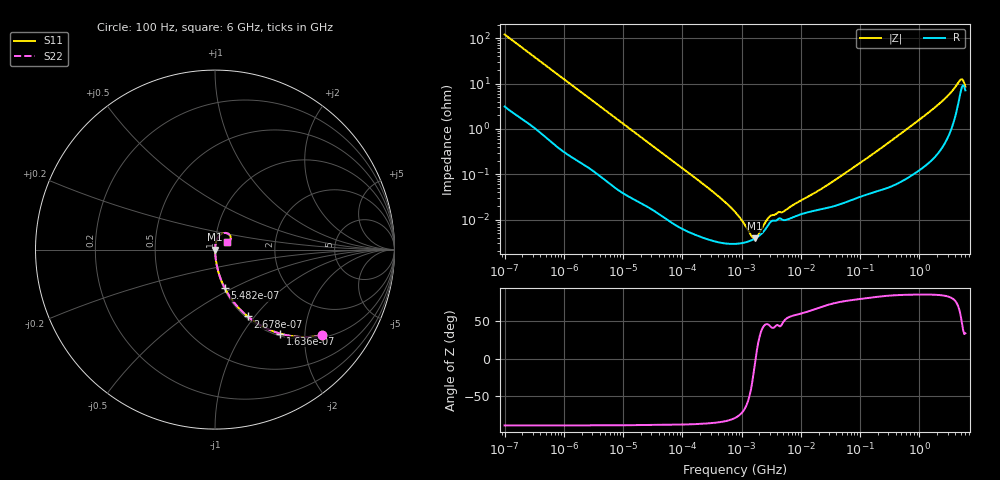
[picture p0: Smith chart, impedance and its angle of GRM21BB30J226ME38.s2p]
!Murata Part Number: GRM21BB30J226ME38
!These Parameters are Measured in Series Mode Connection
!  o--ll--o
!Port1  Port2
!  o------o
!Operation Temp=20[C], DC Bias Voltage=0[V]
!Freq. Start=100[Hz] Stop=6[GHz], 401[Steps]
# Hz S RI R 50
!Freq.(Hz) S11(Real) S11(Imag) S21(Real) S21(Imag) S12(Real) S12(Imag) S22(Real) S22(Imag)
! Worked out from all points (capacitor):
!   401 points, 100 Hz to 6 GHz, reference 50 ohm
!   read as one part in series: C = 13.1 uF near 109.4 Hz
!   lowest |Z| = 3.85 mohm at 1.658 MHz (marker M1)
!   series resonance near 1.725 MHz, so ESL is about 650 pH
!   S11 on the Smith chart (normalised r, x): 100 Hz: 1.06, -2.43; 163.6 Hz: 1.04, -1.49; 267.8 Hz: 1.03, -0.92; 548.2 Hz: 1.01, -0.46; 6 GHz: 1.14, +0.10
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100  0.5936 -0.4785  0.4064 0.4785  0.4064 0.4785  0.5936 -0.4785
163.6437  0.3619 -0.4676  0.6381 0.4676  0.6381 0.4676  0.3619 -0.4676
267.7924  0.1817 -0.3723  0.8183 0.3723  0.8183 0.3723  0.1817 -0.3723
548.1815  0.0544 -0.2143  0.9456 0.2143  0.9456 0.2143  0.0544 -0.2143
2008.354  0.00572 -0.0629  0.9943 0.0629  0.9943 0.0629  0.00572 -0.0629
40334.87  0.000144 -0.00334  0.9999 0.00334  0.9999 0.00334  0.000144 -0.00334
330836.5  3.41e-05 -0.000409  1 0.000409  1 0.000409  3.41e-05 -0.000409
774596.7  2.93e-05 -0.000146  1 0.000146  1 0.000146  2.93e-05 -0.000146
926525  2.99e-05 -0.000109  1 0.000109  1 0.000109  2.99e-05 -0.000109
1059725  3.08e-05 -8.32e-05  1 8.32e-05  1 8.32e-05  3.08e-05 -8.32e-05
1658239  3.8e-05 -6.46e-06  1 6.46e-06  1 6.46e-06  3.8e-05 -6.46e-06
2594782  6.45e-05 6.74e-05  0.9999 -6.74e-05  0.9999 -6.74e-05  6.45e-05 6.74e-05
3245845  9.4e-05 8.31e-05  0.9999 -8.31e-05  0.9999 -8.31e-05  9.4e-05 8.31e-05
5311619  9.76e-05 0.000122  0.9999 -0.000122  0.9999 -0.000122  9.76e-05 0.000122
1.555665e7  0.000154 0.000329  0.9998 -0.000329  0.9998 -0.000329  0.000154 0.000329
4.165952e7  0.00021 0.000789  0.9998 -0.000789  0.9998 -0.000789  0.00021 0.000789
3.124326e8  0.000546 0.00512  0.9995 -0.00512  0.9995 -0.00512  0.000546 0.00512
2.048624e9  0.00396 0.0334  0.996 -0.0334  0.996 -0.0334  0.00396 0.0334
3.205649e9  0.0109 0.0569  0.9891 -0.0569  0.9891 -0.0569  0.0109 0.0569
4.796499e9  0.0577 0.0931  0.9423 -0.0931  0.9423 -0.0931  0.0577 0.0931
5.245841e9  0.0846 0.0789  0.9154 -0.0789  0.9154 -0.0789  0.0846 0.0789
6e9  0.0682 0.0418  0.9318 -0.0418  0.9318 -0.0418  0.0682 0.0418
